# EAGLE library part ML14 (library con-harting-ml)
HARTING
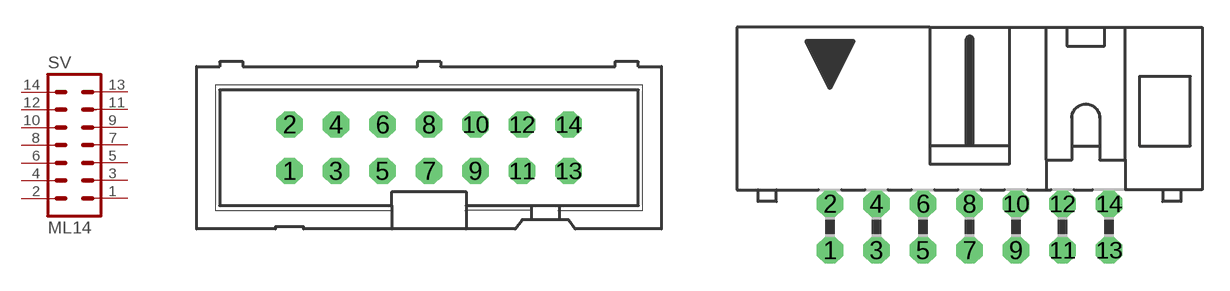
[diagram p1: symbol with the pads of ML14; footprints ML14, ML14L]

Designator prefix SV

## ML14 (OC_FARNELL: unknown; OC_NEWARK: unknown)  [ML14]
1  1  pas
2  2  pas
3  3  pas
4  4  pas
5  5  pas
6  6  pas
7  7  pas
8  8  pas
9  9  pas
10  10  pas
11  11  pas
12  12  pas
13  13  pas
14  14  pas

## ML14L (OC_FARNELL: unknown; OC_NEWARK: unknown)  [ML14L]
Pads as for ML14

## ML14-3M (OC_FARNELL: unknown; OC_NEWARK: unknown)  [3M_14]
Pads as for ML14

## ML14-3ML (OC_FARNELL: unknown; OC_NEWARK: unknown)  [3M_14L]
Pads as for ML14

## Footprint ML14 (pad centres in mm)
HARTING
drill 0.914 octagon: 1 -7.62,-1.27; 2 -7.62,1.27; 3 -5.08,-1.27; 4 -5.08,1.27; 5 -2.54,-1.27; 6 -2.54,1.27; 7 0,-1.27; 8 0,1.27; 9 2.54,-1.27; 10 2.54,1.27; 11 5.08,-1.27; 12 5.08,1.27; 13 7.62,-1.27; 14 7.62,1.27

## Footprint ML14L (pad centres in mm)
HARTING
drill 0.914 octagon: 1 -7.62,-1.27; 2 -7.62,1.27; 3 -5.08,-1.27; 4 -5.08,1.27; 5 -2.54,-1.27; 6 -2.54,1.27; 7 0,-1.27; 8 0,1.27; 9 2.54,-1.27; 10 2.54,1.27; 11 5.08,-1.27; 12 5.08,1.27; 13 7.62,-1.27; 14 7.62,1.27

## Footprint 3M_14 (pad centres in mm)
3M
drill 0.813 square: 1 -7.62,-1.27; 2 -7.62,1.27; 3 -5.08,-1.27; 4 -5.08,1.27; 5 -2.54,-1.27; 6 -2.54,1.27; 7 0,-1.27; 8 0,1.27; 9 2.54,-1.27; 10 2.54,1.27; 11 5.08,-1.27; 12 5.08,1.27; 13 7.62,-1.27; 14 7.62,1.27

## Footprint 3M_14L (pad centres in mm)
3M
drill 0.813 square: 1 -7.62,-5.08; 2 -7.62,-2.54; 3 -5.08,-5.08; 4 -5.08,-2.54; 5 -2.54,-5.08; 6 -2.54,-2.54; 7 0,-5.08; 8 0,-2.54; 9 2.54,-5.08; 10 2.54,-2.54; 11 5.08,-5.08; 12 5.08,-2.54; 13 7.62,-5.08; 14 7.62,-2.54
hole 2.54 at -13.538,-3.277
hole 2.54 at 13.538,-3.277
